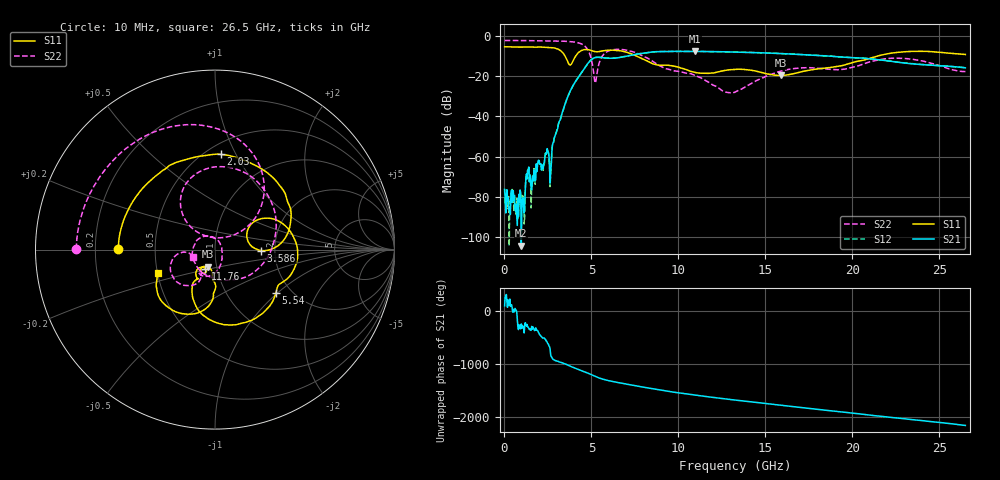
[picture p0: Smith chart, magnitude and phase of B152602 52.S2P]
!  2-Port S-parameters saved by WinCal
! VAR MeasName=S-Parameters (CALIBRATED_DATA) read from VNA (N5242A)
! VAR MeasDate=2016-1-5 16:33:29
! VAR NAME=B152602 52
! VAR FILENAME=B152602 52.S2P
! VAR DATE=2016-1-5 16:33:29
! VAR PHYS_PORTS=1,2
# Hz S DB R 50
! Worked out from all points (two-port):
!   801 points, 10 MHz to 26.5 GHz, reference 50 ohm
!   highest |S21| = -7.67 dB at 10.94 GHz (marker M1); lowest = -104.3 dB at 970.3 MHz (marker M2)
!   |S21| within 3 dB of the highest: 5.254 GHz to 5.515 GHz (261.6 MHz wide, 4.86 % of centre); 6.646 GHz to 19.68 GHz (13.03 GHz wide, 99 % of centre)
!   lowest |S11| = -19.7 dB at 15.87 GHz (marker M3), VSWR 1.23, Z = 45.3 - j8.78 ohm
!   |S11| at or under -10 dB: 3.484 GHz to 4.094 GHz (609.9 MHz wide, 16.1 % of centre); 7.59 GHz to 21.46 GHz (13.87 GHz wide, 95.5 % of centre)
!   |S22| runs from -28.3 to -2.2 dB; largest |S21 - S12| = 0.0028
!   S11 on the Smith chart (normalised r, x): 10 MHz: 0.30, +0.00; 2.03 GHz: 0.59, +0.87; 3.586 GHz: 1.69, -0.02; 5.54 GHz: 1.67, -0.98; 11.76 GHz: 0.88, -0.19; 26.5 GHz: 0.50, -0.15
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1e7  -5.38 179.5  -76.33 101.4  -76.24 -110.0  -2.24 179.8
9.702625e8  -5.55 136.2  -104.27 121.5  -80.64 75.4  -2.29 165.0
1.3345e9  -5.51 120.1  -66.77 63.0  -66.88 74.2  -2.32 159.2
1.632512e9  -5.57 105.7  -69.80 65.6  -69.39 65.0  -2.35 154.4
2.029862e9  -5.49 86.6  -63.81 -84.4  -63.77 -81.2  -2.39 147.7
2.692112e9  -5.76 51.4  -64.08 -134.7  -63.71 -135.4  -2.46 135.4
2.890788e9  -6.00 38.8  -50.10 155.7  -50.06 155.1  -2.49 131.2
3.58615e9  -11.78 -1.2  -31.41 74.2  -31.41 74.2  -2.69 113.8
4.447075e9  -7.19 11.5  -17.98 -41.8  -17.97 -41.7  -4.03 78.1
4.844425e9  -6.88 -14.1  -13.16 -93.4  -13.16 -93.3  -7.76 48.3
5.208662e9  -7.79 -28.1  -10.76 -147.2  -10.75 -147.1  -23.44 75.6
5.539788e9  -7.59 -35.6  -10.70 171.7  -10.69 171.8  -11.31 132.1
7.062962e9  -8.18 -94.9  -10.00 64.1  -9.95 64.1  -7.15 54.4
8.851038e9  -14.53 -120.5  -7.78 -40.0  -7.75 -40.1  -14.51 -64.4
1.093712e10  -18.08 -127.8  -7.67 -139.4  -7.67 -139.3  -19.55 141.8
1.176494e10  -18.55 -116.8  -7.78 -174.4  -7.76 -174.3  -23.08 99.1
1.3255e10  -16.65 -116.3  -8.01 126.3  -7.99 126.2  -27.90 -13.2
1.587089e10  -19.66 -112.8  -8.76 27.8  -8.76 28.0  -17.58 -90.9
1.769208e10  -16.79 -96.0  -9.53 -38.0  -9.50 -37.8  -15.88 -121.7
1.957949e10  -14.34 -89.4  -10.62 -105.2  -10.57 -105.1  -16.47 -119.9
2.209604e10  -8.75 -105.1  -12.49 163.3  -12.40 163.1  -11.19 -137.8
2.65e10  -9.21 -157.4  -15.85 7.4  -15.85 7.1  -17.72 -160.6
